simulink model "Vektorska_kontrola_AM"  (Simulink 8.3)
settings: Solver=ode3  StartTime=0  StopTime=Tfinalno  FixedStep=Tsim  RelTol=1e-3
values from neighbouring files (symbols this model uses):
  A1 = [-Rsigma/Lsigma 0 Lm/(Tr*Lr*Lsigma) 0; 0 -Rsigma/Lsigma 0 Lm/(Tr*Lr*Lsigma); Lm/Tr 0 -1/Tr 0; 0 Lm/Tr 0 -1/Tr]    [Vektorska_kontrola_AM_parametri.m]
  A2 = [0 1 0 0; -1 0 0 0; 0 0 0 1; 0 0 -1 0]    [Vektorska_kontrola_AM_parametri.m]
  A3 = [0 0 0 Lm/(Lr*Lsigma); 0 0 -Lm/(Lr*Lsigma) 0; 0 0 0 -1; 0 0 1 0]    [Vektorska_kontrola_AM_parametri.m]
  B = [1/Lsigma 0; 0 1/Lsigma; 0 0; 0 0]    [Vektorska_kontrola_AM_parametri.m]
  fdq = 50    [Vektorska_kontrola_AM_parametri.m]
  flux_bazno_dsp = Vbazno_dsp/wbazno_dsp    (= 0.0641171388295)    [Vektorska_kontrola_AM_parametri.m]
  fpwm = 20000    [Vektorska_kontrola_AM_parametri.m]
  Ibazno_dsp = Imax    (= 720)    [Vektorska_kontrola_AM_parametri.m]
  Imax = 720    [Vektorska_kontrola_AM_parametri.m]
  Isd_max = 100    [Vektorska_kontrola_AM_parametri.m]
  Isd_min = 12    [Vektorska_kontrola_AM_parametri.m]
  Isd_nom_fazno = sqrt(2)*25    [Vektorska_kontrola_AM_parametri.m]
  Isd_rel = Isd_nom_fazno/Ibazno_dsp    [Vektorska_kontrola_AM_parametri.m]
  Isq_rel = Isq_nom_fazno/Ibazno_dsp    [Vektorska_kontrola_AM_parametri.m]
  J = 0.001    [Vektorska_kontrola_AM_parametri.m]
  k_foc = 1.1    [Vektorska_kontrola_AM_parametri.m]
  k_rs = 1    [Vektorska_kontrola_AM_parametri.m]
  Ki_i = Kp_i* TkrozTsigma    [Vektorska_kontrola_AM_parametri.m]
  Ki_w = 50*0.03512/K    [Vektorska_kontrola_AM_parametri.m]
  Kp_i = (1-exp(-lambda*T))/(Kps*(exp(T/Tsigma)-1)*(1+n*(1-exp(-lambda*T))))    [Vektorska_kontrola_AM_parametri.m]
  Kp_w = 4*0.2027/K    [Vektorska_kontrola_AM_parametri.m]
  Lm = 0.00094    [Vektorska_kontrola_AM_parametri.m]
  Lm_rel = Lm/L_bazno_dsp    (= 10.55568)    [Vektorska_kontrola_AM_parametri.m]
  Lr = Lxr+Lm    (= 0.000968)    [Vektorska_kontrola_AM_parametri.m]
  Lsigma = Ls*sigm    (= 5.51900826446e-05)    [Vektorska_kontrola_AM_parametri.m]
  Lsigma_rel = Lsigma/L_bazno_dsp    (= 0.619754097415)    [Vektorska_kontrola_AM_parametri.m]
  Mopt = 2    [Vektorska_kontrola_AM_parametri.m]
  n_fw = 3500    [Vektorska_kontrola_AM_parametri.m]
  p = 2    [Vektorska_kontrola_AM_parametri.m]
  Rs_rel = Rs/R_bazno_dsp    (= 0.0284680851064)    [Vektorska_kontrola_AM_parametri.m]
  t1_step = 2    [Vektorska_kontrola_AM_parametri.m]
  t2_step = 4    [Vektorska_kontrola_AM_parametri.m]
  topt = 1    [Vektorska_kontrola_AM_parametri.m]
  Tpwm = 1/fpwm    (= 5e-05)    [Vektorska_kontrola_AM_parametri.m]
  Tpwm_SV = 1000    [Vektorska_kontrola_AM_parametri.m]
  Tr = Lr/Rr    (= 0.175680580762)    [Vektorska_kontrola_AM_parametri.m]
  TROUGAO_ZVEZDA = 0    [Vektorska_kontrola_AM_parametri.m]
  Tsim = Tpwm/16    (= 3.125e-06)    [Vektorska_kontrola_AM_parametri.m]
  Twreg1 = 320*Tsim    (= 0.001)    [Vektorska_kontrola_AM_parametri.m]
  ugao_dq = 0    [Vektorska_kontrola_AM_parametri.m]
  Vbazno_dsp = Vmax    (= 112.8)    [Vektorska_kontrola_AM_parametri.m]
  Vd = 30    [Vektorska_kontrola_AM_parametri.m]
  Vdc = 48    [Vektorska_kontrola_AM_parametri.m]
  Vq = 0    [Vektorska_kontrola_AM_parametri.m]
  wb1 = 3431    [Vektorska_kontrola_AM_parametri.m]
  wbazno_dsp = 879.64*2    (= 1759.28)    [Vektorska_kontrola_AM_parametri.m]
  wgr = 2*pi()*fgr    [Vektorska_kontrola_AM_parametri.m]
undefined symbols (not defined in the file or in its folder): DiscIntNeverNeededParam
libraries: simulink_extras x4, simulink x2

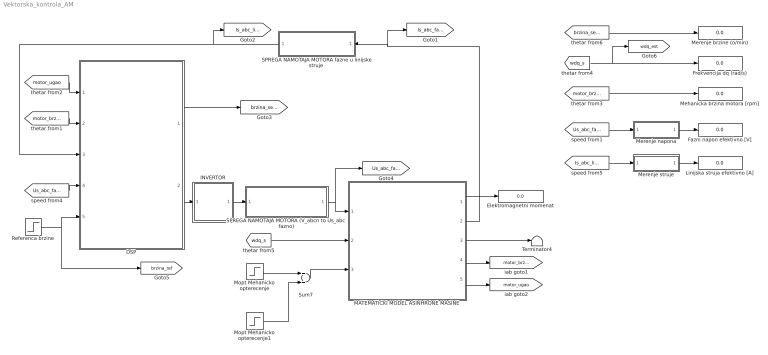
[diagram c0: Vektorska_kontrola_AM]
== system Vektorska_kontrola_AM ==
  DSP : Subsystem
  Elektromagnetni momenat : Display
  Fazni napon efektivno [V] : Display
  Frekvencija dq (rad/s) : Display
  INVERTOR : Subsystem
  Linijska struja efektivno [A] : Display
  MATEMATICKI MODEL ASINHRONE MASINE : Subsystem
  Mehanicka brzina motora [rpm] : Display
  Merenje brzine (o/min) : Display
  Merenje napona : Subsystem
  Merenje struje : Subsystem
  Mopt Mehanicko opterecenje : Step  Time=topt  After=Mopt  SampleTime=Tsim
  Mopt Mehanicko opterecenje1 : Step  Time=3*topt  After=Mopt  SampleTime=Tsim
  Referenca brzine : Step  Time=0.5  After=300  SampleTime=Tsim
  SPREGA NAMOTAJA MOTORA (V_abcn to Us_abc  fazno) : Subsystem
  "SPREGA NAMOTAJA MOTORA fazne u linijske struje " : Subsystem
  Sum7 : Sum  SampleTime=Tsim
  Terminator4 : Terminator
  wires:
  [wdq_s] -> MATEMATICKI MODEL ASINHRONE MASINE/2(W_dq)
  MATEMATICKI MODEL ASINHRONE MASINE/1(M_el) -> Elektromagnetni momenat/1
  Merenje napona/1(Us_eff) -> Fazni napon efektivno [V]/1
  Merenje struje/1(Is_eff) -> Linijska struja efektivno [A]/1
  [Is_abc_linijsko] -> Merenje struje/1(Is_abc)
  [Us_abc_fazno] -> Merenje napona/1(Us_abc)
  [motor_brzina] -> Mehanicka brzina motora [rpm]/1
  "SPREGA NAMOTAJA MOTORA fazne u linijske struje "/1("Is_abc  invertor ") -> [Is_abc_linijsko], DSP/3(Is_abc (linijsko))
  [motor_brzina] -> DSP/2(Mehanicka brzina  [o/min])
  [motor_ugao] -> DSP/1(Ugao el [rad])
  [Us_abc_fazno] -> DSP/4(Us_abc (fazno))
  INVERTOR/1(U_abcn) -> SPREGA NAMOTAJA MOTORA (V_abcn to Us_abc  fazno)/1(Uabc_prema_n)
  DSP/2(V_abc ref) -> INVERTOR/1(ABC)
  SPREGA NAMOTAJA MOTORA (V_abcn to Us_abc  fazno)/1(Us_abc_fazno) -> MATEMATICKI MODEL ASINHRONE MASINE/1(Us_abc), [Us_abc_fazno]
  [wdq_s] -> [wdq_est], Frekvencija dq (rad/s)/1
  DSP/1(Brzina (est) Senzor) -> [brzina_senzor]
  [brzina_senzor] -> Merenje brzine (o/min)/1
  MATEMATICKI MODEL ASINHRONE MASINE/2(Is_abc) -> "SPREGA NAMOTAJA MOTORA fazne u linijske struje "/1(Is_abc fazno), [Is_abc_fazno]
  Referenca brzine/1 -> DSP/5(Referenca brzine), [brzina_ref]
  MATEMATICKI MODEL ASINHRONE MASINE/5(ugao rot_el) -> [motor_ugao]
  MATEMATICKI MODEL ASINHRONE MASINE/4(Brzina meh [o/min]) -> [motor_brzina]
  Mopt Mehanicko opterecenje/1 -> Sum7/1
  Mopt Mehanicko opterecenje1/1 -> Sum7/2
  Sum7/1 -> MATEMATICKI MODEL ASINHRONE MASINE/3(Mopt)
  MATEMATICKI MODEL ASINHRONE MASINE/3(Wr_el) -> Terminator4/1

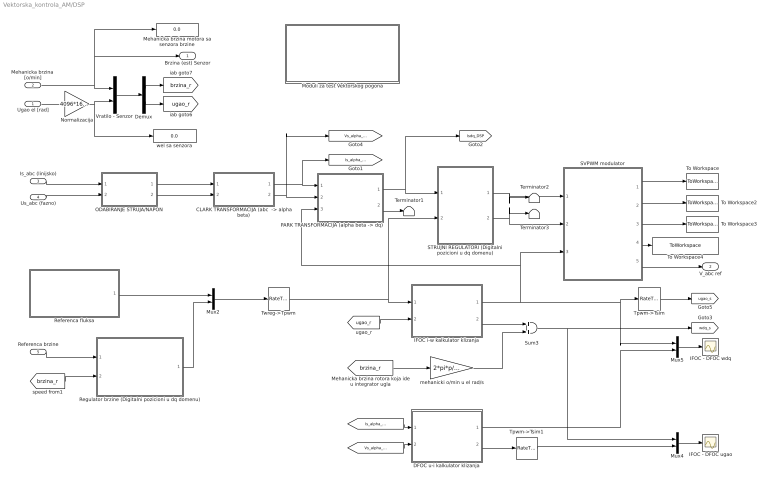
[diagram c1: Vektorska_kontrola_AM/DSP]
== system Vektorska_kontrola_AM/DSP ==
  Ugao el [rad] : Inport
  Mehanicka brzina  [o/min] : Inport  Port=2
  Is_abc (linijsko) : Inport  Port=3
  Us_abc (fazno) : Inport  Port=4
  Referenca brzine : Inport  Port=5
  "CLARK TRANSFORMACIJA (abc  -> alpha beta)" : Subsystem
  DFOC u-i kalkulator klizanja : Subsystem
  Demux : Demux  Outputs=2
  IFOC - DFOC ugao : Scope
  IFOC - DFOC wdq : Scope
  IFOC i-w kalkulator klizanja : Subsystem
  Mehanicka brzina motora sa senzora brzine : Display
  Moduli za test Vektorskog pogona : Subsystem
  Mux2 : Mux  Inputs=2
  Mux4 : Mux  Inputs=2
  Mux5 : Mux  Inputs=2
  Normalizacija : Gain  Gain=4096*16/(2*pi)  SampleTime=Tsim
  ODABIRANJE STRUJA/NAPON : Subsystem
  "PARK TRANSFORMACIJA (alpha beta -> dq)" : Subsystem
  Referenca fluksa : Subsystem
  Regulator brzine (Digitalni pozicioni u dq domenu) : Subsystem
  STRUJNI REGULATORI (Digitalni pozicioni u dq domenu) : Subsystem
  SVPWM modulator : Subsystem
  Sum3 : Sum  SampleTime=Tsim
  Terminator1 : Terminator
  Terminator2 : Terminator
  Terminator3 : Terminator
  To Workspace : ToWorkspace  VariableName=ugao  SampleTime=-1
  To Workspace2 : ToWorkspace  VariableName=BrojSektora  SampleTime=-1
  To Workspace3 : ToWorkspace  VariableName=T1T2T0  SampleTime=-1
  To Workspace4 : ToWorkspace  VariableName=LONG_MIDDLE_SHORT  SampleTime=-1
  Tpwm->Tsim : RateTransition  OutPortSampleTime=Tsim
  Tpwm->Tsim1 : RateTransition  OutPortSampleTime=Tsim
  Twreg->Tpwm : RateTransition  OutPortSampleTime=Tpwm
  Vratilo - Senzor : Mux  Inputs=2
  mehanicki o/min u el rad/s : Gain  Gain=2*pi*p/60  SampleTime=Tsim
  wel sa senzora : Display
  Brzina (est) Senzor : Outport
  V_abc ref : Outport  Port=2
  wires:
  Ugao el [rad]/1 -> Normalizacija/1
  Mehanicka brzina  [o/min]/1 -> Vratilo - Senzor/1, Mehanicka brzina motora sa senzora brzine/1, Brzina (est) Senzor/1
  Vratilo - Senzor/1 -> Demux/1
  Demux/1 -> [brzina_r]
  Normalizacija/1 -> Vratilo - Senzor/2, wel sa senzora/1
  ODABIRANJE STRUJA/NAPON/1(Is_abc DSP) -> "CLARK TRANSFORMACIJA (abc  -> alpha beta)"/1(Is_abc)
  ODABIRANJE STRUJA/NAPON/2(Us_abc DSP) -> "CLARK TRANSFORMACIJA (abc  -> alpha beta)"/2(Us_abc)
  "PARK TRANSFORMACIJA (alpha beta -> dq)"/2(Us_dq) -> Terminator1/1
  "CLARK TRANSFORMACIJA (abc  -> alpha beta)"/1(Is_alpha_beta) -> [Is_alpha_beta_DSP], "PARK TRANSFORMACIJA (alpha beta -> dq)"/1(Is_alpha_beta)
  "CLARK TRANSFORMACIJA (abc  -> alpha beta)"/2(Us_alpha_beta) -> [Vs_alpha_beta_DSP], "PARK TRANSFORMACIJA (alpha beta -> dq)"/2(Us_alpha_beta)
  Regulator brzine (Digitalni pozicioni u dq domenu)/1(Referenca momenta) -> Mux2/2
  Is_abc (linijsko)/1 -> ODABIRANJE STRUJA/NAPON/1(Is_abc)
  [brzina_r] -> mehanicki o/min u el rad/s/1
  [brzina_r] -> Regulator brzine (Digitalni pozicioni u dq domenu)/2(nr)
  Referenca brzine/1 -> Regulator brzine (Digitalni pozicioni u dq domenu)/1(nr_ref)
  SVPWM modulator/5(Tabc) -> V_abc ref/1
  "PARK TRANSFORMACIJA (alpha beta -> dq)"/1(Is_dq) -> [Isdq_DSP], STRUJNI REGULATORI (Digitalni pozicioni u dq domenu)/1(Is_dq)
  Us_abc (fazno)/1 -> ODABIRANJE STRUJA/NAPON/2(Us_abc)
  Mux2/1 -> Twreg->Tpwm/1
  SVPWM modulator/4(LONG_MIDDLE_SHORT) -> To Workspace4/1
  SVPWM modulator/3(T1T2T0) -> To Workspace3/1
  SVPWM modulator/2(BrojSektora) -> To Workspace2/1
  SVPWM modulator/1(ugao) -> To Workspace/1
  Referenca fluksa/1(Flux_referenca) -> Mux2/1
  Demux/2 -> [ugao_r]
  Tpwm->Tsim/1 -> [ugao_s]
  STRUJNI REGULATORI (Digitalni pozicioni u dq domenu)/1(Vds_ref) -> SVPWM modulator/1(Vsd_ref), Terminator2/1
  STRUJNI REGULATORI (Digitalni pozicioni u dq domenu)/2(Vqs_ref) -> SVPWM modulator/2(Vsq_ref), Terminator3/1
  IFOC i-w kalkulator klizanja/1(ugao) -> "PARK TRANSFORMACIJA (alpha beta -> dq)"/3(ugao_DSP), SVPWM modulator/3(ugao dq), Mux5/1, Tpwm->Tsim/1
  IFOC i-w kalkulator klizanja/2(w_k) -> Sum3/1
  Mux4/1 -> IFOC - DFOC ugao/1
  DFOC u-i kalkulator klizanja/2(w_dq) -> Tpwm->Tsim1/1
  Sum3/1 -> [wdq_s], Mux4/1
  Mux5/1 -> IFOC - DFOC wdq/1
  Twreg->Tpwm/1 -> STRUJNI REGULATORI (Digitalni pozicioni u dq domenu)/2(Is_dq_ref), IFOC i-w kalkulator klizanja/1(Is_dq_ref)
  [ugao_r] -> IFOC i-w kalkulator klizanja/2(ugao rotor)
  mehanicki o/min u el rad/s/1 -> Sum3/2
  [Is_alpha_beta_DSP] -> DFOC u-i kalkulator klizanja/1(Is_alpha_beta)
  [Vs_alpha_beta_DSP] -> DFOC u-i kalkulator klizanja/2(Us_alpha_beta)
  Tpwm->Tsim1/1 -> Mux4/2
  DFOC u-i kalkulator klizanja/1(ugao) -> Mux5/2

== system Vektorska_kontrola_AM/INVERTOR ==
  ABC : Inport
  Pojacanje : Gain  Gain=2/Tpwm_SV
  Proizvod : Product
  U_abcn : Outport  InitialOutput=0
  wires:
  Pojacanje/1 -> U_abcn/1
  [DC_napon] -> Proizvod/2
  ABC/1 -> Proizvod/1
  Proizvod/1 -> Pojacanje/1

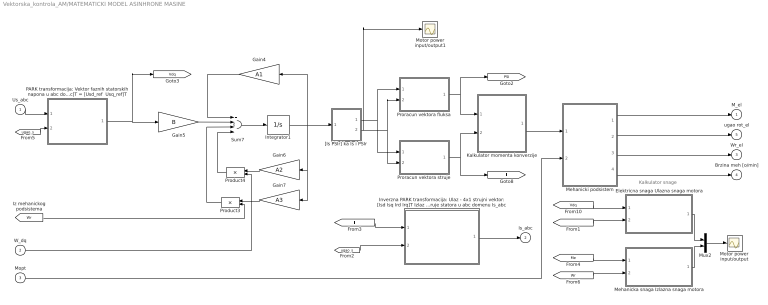
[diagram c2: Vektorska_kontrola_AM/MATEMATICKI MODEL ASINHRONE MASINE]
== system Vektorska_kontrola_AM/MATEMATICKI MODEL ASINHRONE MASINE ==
  note: Kalkulator snage
  Us_abc : Inport
  W_dq : Inport  Port=2
  Mopt : Inport  Port=3
  Elektricna snaga Ulazna snaga motora : Subsystem
  Gain4 : Gain  Gain=A1  Multiplication=Matrix(K*u) (u vector)  SampleTime=Tsim
  Gain5 : Gain  Gain=B  Multiplication=Matrix(K*u) (u vector)  SampleTime=Tsim
  Gain6 : Gain  Gain=A2  Multiplication=Matrix(K*u) (u vector)  SampleTime=Tsim
  Gain7 : Gain  Gain=A3  Multiplication=Matrix(K*u) (u vector)  SampleTime=Tsim
  Integrator1 : Integrator  InitialCondition=[0,0,0,0]
  Inverzna PARK transformacija: Ulaz - 4x1 strujni vektor: [Isd Isq Ird Irq]T Izlaz - vektor struje statora u abc domenu Is_abc : Subsystem
  Kalkulator momenta konverzije : Subsystem
  Mehanicka snaga Izlazna snaga motora : Subsystem
  Mehanicki podsistem : Subsystem
  Motor power input/output : Scope
  Motor power input/output1 : Scope
  Mux2 : Mux  Inputs=2
  PARK transformacija: Vektor faznih statorskih napona u abc domenu u vektor napona u dq referentnom sistemu - [Usa  Usb Usc]T = [Usd_ref  Usq_ref]T : Subsystem
  Product3 : Product  SampleTime=Tsim
  Product4 : Product  SampleTime=Tsim
  Proracun vektora fluksa : Subsystem
  Proracun vektora struje : Subsystem
  Sum7 : Sum  Inputs=++++  SampleTime=Tsim
  "[Is PSIr] ka Is i PSIr" : Subsystem
  M_el : Outport  InitialOutput=0
  Is_abc : Outport  Port=2  InitialOutput=0
  Wr_el : Outport  Port=3  InitialOutput=0
  Brzina meh [o/min] : Outport  Port=4  InitialOutput=0
  ugao rot_el : Outport  Port=5  InitialOutput=0
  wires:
  Us_abc/1 -> PARK transformacija: Vektor faznih statorskih napona u abc domenu u vektor napona u dq referentnom sistemu - [Usa  Usb Usc]T = [Usd_ref  Usq_ref]T/1(Us_abc)
  [ugao_s] -> PARK transformacija: Vektor faznih statorskih napona u abc domenu u vektor napona u dq referentnom sistemu - [Usa  Usb Usc]T = [Usd_ref  Usq_ref]T/2(ugao_dq)
  Integrator1/1 -> Gain4/1, Gain7/1, Gain6/1, "[Is PSIr] ka Is i PSIr"/1(X1)
  [Wr] -> Product3/2
  Product3/1 -> Sum7/3
  Gain7/1 -> Product3/1
  Gain6/1 -> Product4/1
  Sum7/1 -> Integrator1/1
  Gain4/1 -> Sum7/1
  Gain5/1 -> Sum7/2
  W_dq/1 -> Product4/2
  [ugao_s] -> Inverzna PARK transformacija: Ulaz - 4x1 strujni vektor: [Isd Isq Ird Irq]T Izlaz - vektor struje statora u abc domenu Is_abc/2(ugao_dq)
  [I] -> Inverzna PARK transformacija: Ulaz - 4x1 strujni vektor: [Isd Isq Ird Irq]T Izlaz - vektor struje statora u abc domenu Is_abc/1(I)
  PARK transformacija: Vektor faznih statorskih napona u abc domenu u vektor napona u dq referentnom sistemu - [Usa  Usb Usc]T = [Usd_ref  Usq_ref]T/1(Us_dq) -> Gain5/1, [Vdq]
  Inverzna PARK transformacija: Ulaz - 4x1 strujni vektor: [Isd Isq Ird Irq]T Izlaz - vektor struje statora u abc domenu Is_abc/1(Is_abc) -> Is_abc/1
  [I] -> Elektricna snaga Ulazna snaga motora/2(Is_dq)
  Elektricna snaga Ulazna snaga motora/1(Pel) -> Mux2/1
  [Me] -> Mehanicka snaga Izlazna snaga motora/1(Me)
  [Wr] -> Mehanicka snaga Izlazna snaga motora/2(Wr)
  Mux2/1 -> Motor power input/output/1
  Mehanicka snaga Izlazna snaga motora/1(Pmeh) -> Mux2/2
  [Vdq] -> Elektricna snaga Ulazna snaga motora/1(Vs_dq)
  Product4/1 -> Sum7/4
  "[Is PSIr] ka Is i PSIr"/1(Is) -> Proracun vektora struje/1(Is), Proracun vektora fluksa/1(Is)
  "[Is PSIr] ka Is i PSIr"/2(PSIr) -> Motor power input/output1/1, Proracun vektora struje/2(PSIr), Proracun vektora fluksa/2(PSIr)
  Proracun vektora fluksa/1(PSI) -> [PSI], Kalkulator momenta konverzije/1(PSI)
  Proracun vektora struje/1(I) -> [I], Kalkulator momenta konverzije/2(I)
  Kalkulator momenta konverzije/1(Me) -> Mehanicki podsistem/1(Mel)
  Mopt/1 -> Mehanicki podsistem/2(Mopt)
  Mehanicki podsistem/1(Me) -> M_el/1
  Mehanicki podsistem/2(ugao rot_el) -> ugao rot_el/1
  Mehanicki podsistem/3(Wr_el) -> Wr_el/1
  Mehanicki podsistem/4(Brzina meh [o/min]) -> Brzina meh [o/min]/1

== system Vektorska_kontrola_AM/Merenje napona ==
  Us_abc : Inport
  Mux : Mux  Inputs=2
  Us_alfa : Fcn  Expr=(2/3)*(u[1]-(u[2]+u[3])/2)  SampleTime=Tsim
  Us_amplituda : Fcn  Expr=sqrt(u[1]^2+u[2]^2)  SampleTime=Tsim
  Us_beta : Fcn  Expr=(u[2]-u[3])/sqrt(3)  SampleTime=Tsim
  Us_eff : Outport
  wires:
  Us_abc/1 -> Us_beta/1, Us_alfa/1
  Us_alfa/1 -> Mux/1
  Us_beta/1 -> Mux/2
  Mux/1 -> Us_amplituda/1
  Us_amplituda/1 -> Us_eff/1

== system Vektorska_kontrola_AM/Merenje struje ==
  Is_abc : Inport
  Is_alfa : Fcn  Expr=(2/3)*(u[1]-(u[2]+u[3])/2)  SampleTime=Tsim
  Is_amplituda : Fcn  Expr=sqrt(u[1]^2+u[2]^2)/sqrt(2)  SampleTime=Tsim
  Is_beta : Fcn  Expr=(u[2]-u[3])/sqrt(3)  SampleTime=Tsim
  Mux : Mux  Inputs=2
  Is_eff : Outport
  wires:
  Is_amplituda/1 -> Is_eff/1
  Mux/1 -> Is_amplituda/1
  Is_beta/1 -> Mux/2
  Is_alfa/1 -> Mux/1
  Is_abc/1 -> Is_alfa/1, Is_beta/1

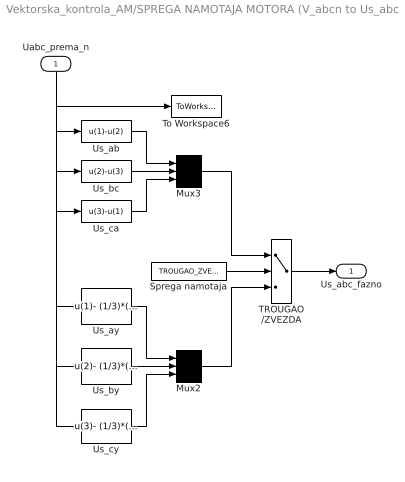
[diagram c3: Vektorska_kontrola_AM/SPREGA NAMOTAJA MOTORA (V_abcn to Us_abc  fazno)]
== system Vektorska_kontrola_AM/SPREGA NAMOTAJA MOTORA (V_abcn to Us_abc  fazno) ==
  Uabc_prema_n : Inport
  Mux2 : Mux  Inputs=3
  Mux3 : Mux  Inputs=3
  Sprega namotaja : Constant  Value=TROUGAO_ZVEZDA  SampleTime=Tsim
  TROUGAO /ZVEZDA : Switch  Threshold=0.1  SampleTime=Tsim
  To Workspace6 : ToWorkspace  VariableName=U_abc_n  SampleTime=Tsim
  Us_ab : Fcn  Expr=u(1)-u(2)  SampleTime=Tsim
  Us_ay : Fcn  Expr=u(1)- (1/3)*(u(1)+u(2)+u(3))  SampleTime=Tsim
  Us_bc : Fcn  Expr=u(2)-u(3)  SampleTime=Tsim
  Us_by : Fcn  Expr=u(2)- (1/3)*(u(1)+u(2)+u(3))  SampleTime=Tsim
  Us_ca : Fcn  Expr=u(3)-u(1)  SampleTime=Tsim
  Us_cy : Fcn  Expr=u(3)- (1/3)*(u(1)+u(2)+u(3))  SampleTime=Tsim
  Us_abc_fazno : Outport  InitialOutput=0
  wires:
  Uabc_prema_n/1 -> Us_ab/1, Us_bc/1, Us_ca/1, Us_ay/1, Us_cy/1, Us_by/1, To Workspace6/1
  Us_by/1 -> Mux2/2
  Us_cy/1 -> Mux2/3
  Us_ay/1 -> Mux2/1
  Us_ab/1 -> Mux3/1
  Us_bc/1 -> Mux3/2
  Us_ca/1 -> Mux3/3
  Mux3/1 -> TROUGAO /ZVEZDA/1
  Mux2/1 -> TROUGAO /ZVEZDA/3
  TROUGAO /ZVEZDA/1 -> Us_abc_fazno/1
  Sprega namotaja/1 -> TROUGAO /ZVEZDA/2

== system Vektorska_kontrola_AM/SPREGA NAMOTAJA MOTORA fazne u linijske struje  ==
  Is_abc fazno : Inport
  Isa_lin=Isa-Isc : Fcn  Expr=u(1)-u(3)  SampleTime=Tsim
  Isb_lin=Isb-Isa : Fcn  Expr=u(2)-u(1)  SampleTime=Tsim
  Isc_lin=Isc-Isb : Fcn  Expr=u(3)-u(2)  SampleTime=Tsim
  Mux2 : Mux  Inputs=3
  Sprega namotaja : Constant  Value=TROUGAO_ZVEZDA
  TROUGAO/ZVEZDA : Switch  Threshold=0.1  SampleTime=Tsim
  "Is_abc  invertor " : Outport  InitialOutput=0
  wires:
  Isc_lin=Isc-Isb/1 -> Mux2/3
  Isb_lin=Isb-Isa/1 -> Mux2/2
  Isa_lin=Isa-Isc/1 -> Mux2/1
  Is_abc fazno/1 -> Isc_lin=Isc-Isb/1, Isb_lin=Isb-Isa/1, Isa_lin=Isa-Isc/1, TROUGAO/ZVEZDA/3
  TROUGAO/ZVEZDA/1 -> "Is_abc  invertor "/1
  Mux2/1 -> TROUGAO/ZVEZDA/1
  Sprega namotaja/1 -> TROUGAO/ZVEZDA/2

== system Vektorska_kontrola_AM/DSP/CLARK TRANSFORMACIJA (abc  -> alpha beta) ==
  Is_abc : Inport
  Us_abc : Inport  Port=2
  Is_alfa : Fcn  Expr=2/3*(u[1]-(u[2]+u[3])/2)
  Is_beta : Fcn  Expr=(u[2]-u[3])/sqrt(3)
  Mux : Mux  Inputs=2
  Mux1 : Mux  Inputs=2
  Us_alfa : Fcn  Expr=(2/3)*(u[1]-(u[2]+u[3])/2)
  Us_beta : Fcn  Expr=(u[2]-u[3])/sqrt(3)
  Is_alpha_beta : Outport
  Us_alpha_beta : Outport  Port=2
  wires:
  Is_beta/1 -> Mux1/2
  Is_alfa/1 -> Mux1/1
  Mux1/1 -> Is_alpha_beta/1
  Mux/1 -> Us_alpha_beta/1
  Us_beta/1 -> Mux/2
  Us_alfa/1 -> Mux/1
  Us_abc/1 -> Us_beta/1, Us_alfa/1
  Is_abc/1 -> Is_beta/1, Is_alfa/1

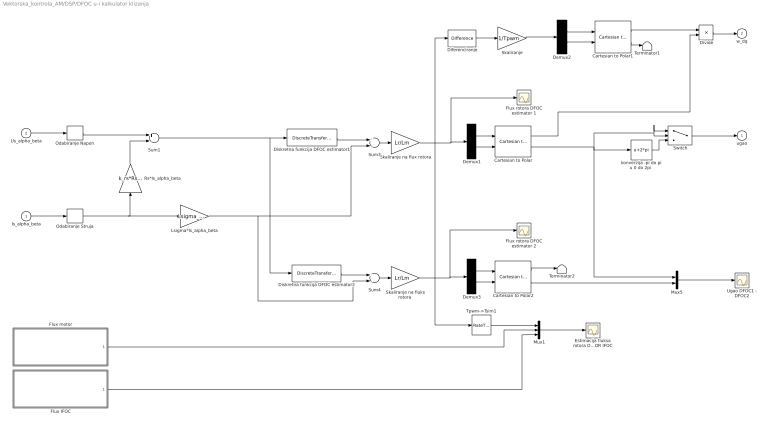
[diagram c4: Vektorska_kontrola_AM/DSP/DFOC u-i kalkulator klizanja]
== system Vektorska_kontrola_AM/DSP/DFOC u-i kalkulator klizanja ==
  Is_alpha_beta : Inport
  Us_alpha_beta : Inport  Port=2
  Cartesian to Polar : simulink_extras/Transformations/Cartesian to Polar
  Cartesian to Polar1 : simulink_extras/Transformations/Cartesian to Polar
  Cartesian to Polar2 : simulink_extras/Transformations/Cartesian to Polar
  Demux1 : Demux  Outputs=2
  Demux2 : Demux  Outputs=2
  Demux3 : Demux  Outputs=2
  Diferenciranje : simulink/Discrete/Difference  ICPrevInput=0.0  OutMin=[]  OutMax=[]  OutDataType=fixdt(1, 16)  OutScaling=2^-10  DoSatur=off
  Diskretna funkcija DFOC estimator1 : DiscreteTransferFcn  Numerator=[wbazno_dsp*Tpwm]  Denominator=[1 -(1-wgr*Tpwm)]  SampleTime=Tpwm
  Diskretna funkcija DFOC estimator2 : DiscreteTransferFcn  Numerator=[wbazno_dsp*Tpwm]  Denominator=[1 -1]  SampleTime=Tpwm
  Divide : Product  Inputs=*/  SampleTime=Tpwm
  Estimacija fluksa rotora DFOC MOTOR IFOC : Scope
  Flux IFOC : Subsystem
  Flux motor : Subsystem
  Flux rotora DFOC estimator 1 : Scope
  Flux rotora DFOC estimator 2 : Scope
  Lsigma*Is_alpha_beta : Gain  Gain=Lsigma_rel  SampleTime=Tpwm
  Mux1 : Mux  Inputs=3
  Mux5 : Mux  Inputs=2
  Odabiranje Napon : ZeroOrderHold  SampleTime=Tpwm
  Odabiranje Struja : ZeroOrderHold  SampleTime=Tpwm
  Rs*Is_alpha_beta : Gain  Gain=k_rs*Rs_rel  SampleTime=Tpwm
  Skaliranje : Gain  Gain=1/Tpwm  SampleTime=Tpwm
  "Skaliranje na fluks rotora " : Gain  Gain=Lr/Lm  SampleTime=Tpwm
  Skaliranje na flux rotora : Gain  Gain=Lr/Lm  SampleTime=Tpwm
  Sum1 : Sum  Inputs=+-  SampleTime=Tpwm
  Sum3 : Sum  Inputs=+-  SampleTime=Tpwm
  Sum4 : Sum  Inputs=+-  SampleTime=Tpwm
  Switch : Switch
  Terminator1 : Terminator
  Terminator2 : Terminator
  Tpwm->Tsim1 : RateTransition  OutPortSampleTime=Tsim
  Ugao DFOC1 - DFOC2 : Scope
  "konverzija -pi do pi u 0 do 2pi " : Fcn  Expr=u+2*pi
  ugao : Outport  InitialOutput=0
  w_dq : Outport  Port=2  InitialOutput=0
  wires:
  Switch/1 -> ugao/1
  Us_alpha_beta/1 -> Odabiranje Napon/1
  Is_alpha_beta/1 -> Odabiranje Struja/1
  Odabiranje Napon/1 -> Sum1/1
  Odabiranje Struja/1 -> Lsigma*Is_alpha_beta/1, Rs*Is_alpha_beta/1
  Rs*Is_alpha_beta/1 -> Sum1/2
  Diskretna funkcija DFOC estimator1/1 -> Sum3/1
  Lsigma*Is_alpha_beta/1 -> Sum4/2, Sum3/2
  Sum3/1 -> Skaliranje na flux rotora/1
  Demux1/1 -> Cartesian to Polar/1
  Demux1/2 -> Cartesian to Polar/2
  Skaliranje na flux rotora/1 -> Flux rotora DFOC estimator 1/1, Demux1/1, Tpwm->Tsim1/1, Diferenciranje/1
  Cartesian to Polar/2 -> "konverzija -pi do pi u 0 do 2pi "/1, Switch/2, Switch/1, Mux5/1
  "konverzija -pi do pi u 0 do 2pi "/1 -> Switch/3
  Skaliranje/1 -> Demux2/1
  Demux2/1 -> Cartesian to Polar1/1
  Demux2/2 -> Cartesian to Polar1/2
  Cartesian to Polar1/1 -> Divide/1
  Divide/1 -> w_dq/1
  Diferenciranje/1 -> Skaliranje/1
  Cartesian to Polar/1 -> Divide/2
  Sum4/1 -> "Skaliranje na fluks rotora "/1
  Diskretna funkcija DFOC estimator2/1 -> Sum4/1
  "Skaliranje na fluks rotora "/1 -> Demux3/1, Flux rotora DFOC estimator 2/1
  Demux3/1 -> Cartesian to Polar2/1
  Demux3/2 -> Cartesian to Polar2/2
  Cartesian to Polar2/2 -> Mux5/2
  Mux5/1 -> Ugao DFOC1 - DFOC2/1
  Mux1/1 -> Estimacija fluksa rotora DFOC MOTOR IFOC/1
  Tpwm->Tsim1/1 -> Mux1/1
  Cartesian to Polar1/2 -> Terminator1/1
  Cartesian to Polar2/1 -> Terminator2/1
  Sum1/1 -> Diskretna funkcija DFOC estimator2/1, Diskretna funkcija DFOC estimator1/1
  Flux motor/1(Flux motor) -> Mux1/2
  Flux IFOC/1(Flux IFOC) -> Mux1/3

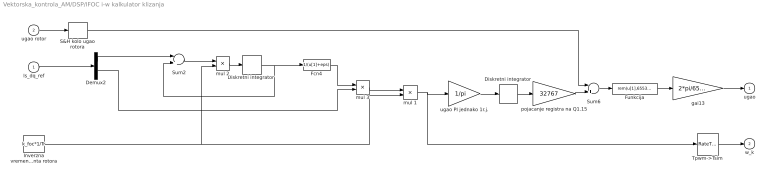
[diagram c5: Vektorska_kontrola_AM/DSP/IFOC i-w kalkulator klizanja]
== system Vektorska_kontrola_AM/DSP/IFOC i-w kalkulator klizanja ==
  Is_dq_ref : Inport
  ugao rotor : Inport  Port=2
  Demux2 : Demux  Outputs=2
  Diskretni integrator : DiscreteIntegrator  SampleTime=Tpwm  ICPrevOutput=DiscIntNeverNeededParam  ICPrevScaledInput=DiscIntNeverNeededParam
  "Diskretni integrator " : DiscreteIntegrator  SampleTime=Tpwm  ICPrevOutput=DiscIntNeverNeededParam  ICPrevScaledInput=DiscIntNeverNeededParam
  Fcn4 : Fcn  Expr=1/(u[1]+eps)  SampleTime=Tpwm
  Funkcija : Fcn  Expr=rem(u[1],65536)  SampleTime=Tpwm
  Inverzna vremenska konstanta rotora : Constant  Value=k_foc*1/Tr  SampleTime=Tpwm
  S&H kolo ugao rotora : ZeroOrderHold  SampleTime=Tpwm
  Sum2 : Sum  Inputs=|+-  SampleTime=Tpwm
  Sum6 : Sum  Inputs=|++  SampleTime=Tpwm
  Tpwm->Tsim : RateTransition  OutPortSampleTime=Tsim
  gai13 : Gain  Gain=2*pi/65535  SampleTime=Tpwm
  mul 1 : Product  SampleTime=Tpwm
  mul 2 : Product  SampleTime=Tpwm
  mul 3 : Product  SampleTime=Tpwm
  pojacanje registra na Q1.15 : Gain  Gain=32767  SampleTime=Tpwm
  ugao PI jednako 1r.j. : Gain  Gain=1/pi  SampleTime=Tpwm
  ugao : Outport  InitialOutput=0
  w_k : Outport  Port=2  InitialOutput=0
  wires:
  Fcn4/1 -> mul 3/1
  Demux2/1 -> Sum2/1
  Demux2/2 -> mul 3/2
  pojacanje registra na Q1.15/1 -> Sum6/2
  Funkcija/1 -> gai13/1
  Sum6/1 -> Funkcija/1
  mul 1/1 -> ugao PI jednako 1r.j./1, Tpwm->Tsim/1
  ugao rotor/1 -> S&H kolo ugao rotora/1
  ugao PI jednako 1r.j./1 -> Diskretni integrator/1
  Diskretni integrator/1 -> pojacanje registra na Q1.15/1
  Is_dq_ref/1 -> Demux2/1
  gai13/1 -> ugao/1
  mul 3/1 -> mul 1/1
  mul 2/1 -> "Diskretni integrator "/1
  "Diskretni integrator "/1 -> Sum2/2, Fcn4/1
  Sum2/1 -> mul 2/1
  Tpwm->Tsim/1 -> w_k/1
  S&H kolo ugao rotora/1 -> Sum6/1
  Inverzna vremenska konstanta rotora/1 -> mul 2/2, mul 1/2

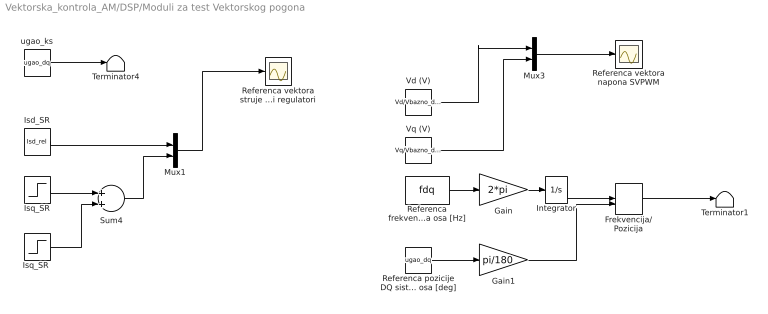
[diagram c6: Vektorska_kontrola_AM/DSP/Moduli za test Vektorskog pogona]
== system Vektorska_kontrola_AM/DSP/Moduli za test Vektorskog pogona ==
  Frekvencija/ Pozicija : ManualSwitch
  Gain : Gain  Gain=2*pi
  Gain1 : Gain  Gain=pi/180
  Integrator : Integrator
  Isd_SR : Constant  Value=Isd_rel  SampleTime=Tpwm
  Isq_SR : Step  Time=t1_step  After=Isq_rel  SampleTime=Tpwm
  "Isq_SR " : Step  Time=t2_step  After=Isq_rel  SampleTime=Tpwm
  Mux1 : Mux  Inputs=2
  Mux3 : Mux  Inputs=2
  Referenca frekvencije DQ sistema osa [Hz] : Constant  Value=fdq
  Referenca pozicije DQ sistema osa [deg] : Constant  Value=ugao_dq
  Referenca vektora napona SVPWM : Scope
  Referenca vektora struje Strujni regulatori : Scope
  Sum4 : Sum  SampleTime=Tpwm
  Terminator1 : Terminator
  Terminator4 : Terminator
  Vd (V) : Constant  Value=Vd/Vbazno_dsp
  Vq (V) : Constant  Value=Vq/Vbazno_dsp
  ugao_ks : Constant  Value=ugao_dq
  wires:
  Gain/1 -> Integrator/1
  Referenca frekvencije DQ sistema osa [Hz]/1 -> Gain/1
  Integrator/1 -> Frekvencija/ Pozicija/1
  Referenca pozicije DQ sistema osa [deg]/1 -> Gain1/1
  Gain1/1 -> Frekvencija/ Pozicija/2
  Isd_SR/1 -> Mux1/1
  Mux1/1 -> Referenca vektora struje Strujni regulatori/1
  Isq_SR/1 -> Sum4/1
  "Isq_SR "/1 -> Sum4/2
  Sum4/1 -> Mux1/2
  Vd (V)/1 -> Mux3/1
  Vq (V)/1 -> Mux3/2
  ugao_ks/1 -> Terminator4/1
  Mux3/1 -> Referenca vektora napona SVPWM/1
  Frekvencija/ Pozicija/1 -> Terminator1/1

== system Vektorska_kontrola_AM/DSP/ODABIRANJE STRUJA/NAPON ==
  Is_abc : Inport
  Us_abc : Inport  Port=2
  S&H kolo naponi : ZeroOrderHold  SampleTime=Tpwm
  S&H kolo struje : ZeroOrderHold  SampleTime=Tpwm
  Skaliranje napona DSP : Gain  Gain=1/ Vbazno_dsp  SampleTime=Tpwm
  Skaliranje struja DSP : Gain  Gain=1/Ibazno_dsp  SampleTime=Tpwm
  linijske u fazne struje - softver - : Subsystem
  Is_abc DSP : Outport  InitialOutput=0
  Us_abc DSP : Outport  Port=2  InitialOutput=0
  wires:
  linijske u fazne struje - softver -/1(Is_abc  fazno) -> Is_abc DSP/1
  Skaliranje struja DSP/1 -> linijske u fazne struje - softver -/1(Is_abc lin)
  Skaliranje napona DSP/1 -> Us_abc DSP/1
  Us_abc/1 -> S&H kolo naponi/1
  Is_abc/1 -> S&H kolo struje/1
  S&H kolo struje/1 -> Skaliranje struja DSP/1
  S&H kolo naponi/1 -> Skaliranje napona DSP/1

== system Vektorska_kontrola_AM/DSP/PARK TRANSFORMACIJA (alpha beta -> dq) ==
  Is_alpha_beta : Inport
  Us_alpha_beta : Inport  Port=2
  ugao_DSP : Inport  Port=3
  ab ->dq1 : Subsystem
  "alpha beta -> dq" : Subsystem
  Is_dq : Outport
  Us_dq : Outport  Port=2
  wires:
  "alpha beta -> dq"/1(Us_dq) -> Us_dq/1
  ab ->dq1/1(Is_dq) -> Is_dq/1
  Us_alpha_beta/1 -> "alpha beta -> dq"/1(Us_alpha_beta)
  Is_alpha_beta/1 -> ab ->dq1/1(Is_alpha_beta)
  ugao_DSP/1 -> ab ->dq1/2(ugao_DSP), "alpha beta -> dq"/2(ugao_DSP)

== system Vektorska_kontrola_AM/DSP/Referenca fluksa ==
  Deljenje : Product  Inputs=*/  SampleTime=Tsim
  Limiter reference fluksa : Subsystem
  Mload_1 : Constant  Value=Isd_nom_fazno  SampleTime=Tsim
  Mload_2 : Constant  Value=n_fw  SampleTime=Tsim
  Odabiranje Flux : ZeroOrderHold  SampleTime=Twreg1
  Referenca fluksa Isd_ref : Scope
  __1 : Gain  Gain=1/Imax  SampleTime=Tsim
  mul 3 : Product  SampleTime=Tsim
  n > n_fw Ulazak u slabljenje polja  Isd_ref = Isd_ref_nom*n/n_fw : Switch  Threshold=n_fw  SampleTime=Tsim
  Flux_referenca : Outport
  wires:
  Mload_1/1 -> __1/1
  Limiter reference fluksa/1("Isd_limit ") -> Odabiranje Flux/1
  Odabiranje Flux/1 -> Flux_referenca/1
  [brzina_r] -> Deljenje/2, n > n_fw Ulazak u slabljenje polja  Isd_ref = Isd_ref_nom*n/n_fw/2
  Mload_2/1 -> Deljenje/1
  __1/1 -> mul 3/2, n > n_fw Ulazak u slabljenje polja  Isd_ref = Isd_ref_nom*n/n_fw/3
  Deljenje/1 -> mul 3/1
  mul 3/1 -> n > n_fw Ulazak u slabljenje polja  Isd_ref = Isd_ref_nom*n/n_fw/1
  n > n_fw Ulazak u slabljenje polja  Isd_ref = Isd_ref_nom*n/n_fw/1 -> Referenca fluksa Isd_ref/1, Limiter reference fluksa/1(Isd_ref)

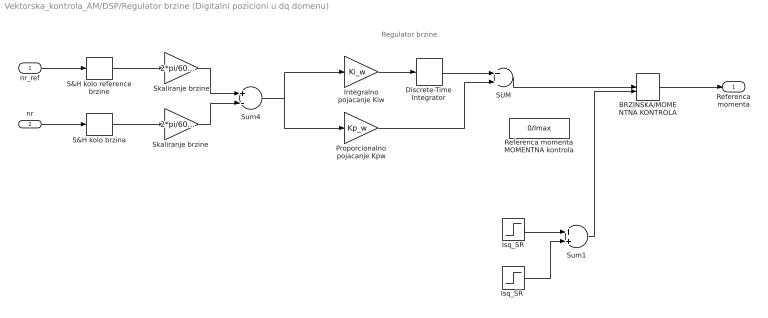
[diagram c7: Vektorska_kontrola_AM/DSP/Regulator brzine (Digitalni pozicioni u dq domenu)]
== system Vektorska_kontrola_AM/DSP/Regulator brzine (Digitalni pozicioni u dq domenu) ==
  note: Regulator brzine
  nr_ref : Inport
  nr : Inport  Port=2
  BRZINSKA/MOMENTNA KONTROLA : ManualSwitch  CurrentSetting=0
  Discrete-Time Integrator : DiscreteIntegrator  SampleTime=Twreg1  ICPrevOutput=DiscIntNeverNeededParam  ICPrevScaledInput=DiscIntNeverNeededParam
  Integralno pojacanje Kiw : Gain  Gain=Ki_w
  Isq_SR : Step  Time=t1_step  After=Isq_rel  SampleTime=Twreg1
  "Isq_SR " : Step  Time=t2_step  After=Isq_rel  SampleTime=Twreg1
  Proporcionalno pojacanje Kpw : Gain  Gain=Kp_w
  Referenca momenta MOMENTNA kontrola : Constant  Value=0/Imax  SampleTime=Twreg1
  S&H kolo brzina : ZeroOrderHold  SampleTime=Twreg1
  S&H kolo reference brzine : ZeroOrderHold  SampleTime=Twreg1
  SUM : Sum  SampleTime=Twreg1
  Skaliranje brzine : Gain  Gain=2*pi/60/wb1
  "Skaliranje brzine " : Gain  Gain=2*pi/60/wb1
  Sum1 : Sum  SampleTime=Twreg1
  Sum4 : Sum  Inputs=+-
  Referenca momenta : Outport  InitialOutput=0
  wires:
  nr/1 -> S&H kolo brzina/1
  nr_ref/1 -> S&H kolo reference brzine/1
  Skaliranje brzine/1 -> Sum4/1
  "Skaliranje brzine "/1 -> Sum4/2
  Sum4/1 -> Proporcionalno pojacanje Kpw/1, Integralno pojacanje Kiw/1
  Integralno pojacanje Kiw/1 -> Discrete-Time Integrator/1
  Discrete-Time Integrator/1 -> SUM/1
  Proporcionalno pojacanje Kpw/1 -> SUM/2
  SUM/1 -> BRZINSKA/MOMENTNA KONTROLA/1
  BRZINSKA/MOMENTNA KONTROLA/1 -> Referenca momenta/1
  S&H kolo reference brzine/1 -> Skaliranje brzine/1
  S&H kolo brzina/1 -> "Skaliranje brzine "/1
  Isq_SR/1 -> Sum1/1
  "Isq_SR "/1 -> Sum1/2
  Sum1/1 -> BRZINSKA/MOMENTNA KONTROLA/2

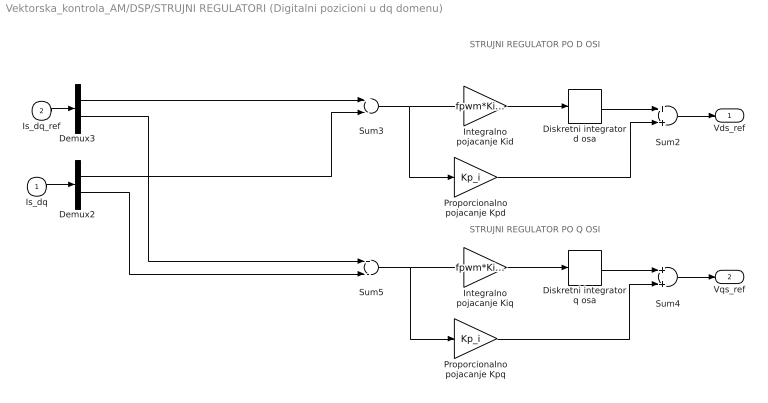
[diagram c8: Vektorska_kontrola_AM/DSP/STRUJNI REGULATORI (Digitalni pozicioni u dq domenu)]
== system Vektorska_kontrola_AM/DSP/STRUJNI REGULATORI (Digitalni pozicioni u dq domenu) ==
  note: STRUJNI REGULATOR PO D OSI
  note: STRUJNI REGULATOR PO Q OSI
  Is_dq : Inport
  Is_dq_ref : Inport  Port=2
  Demux2 : Demux  Outputs=2
  Demux3 : Demux  Outputs=2
  Diskretni integrator d osa : DiscreteIntegrator  SampleTime=Tpwm  ICPrevOutput=DiscIntNeverNeededParam  ICPrevScaledInput=DiscIntNeverNeededParam
  Diskretni integrator q osa : DiscreteIntegrator  SampleTime=Tpwm  ICPrevOutput=DiscIntNeverNeededParam  ICPrevScaledInput=DiscIntNeverNeededParam
  Integralno pojacanje Kid : Gain  Gain=fpwm*Ki_i  SampleTime=Tpwm
  Integralno pojacanje Kiq : Gain  Gain=fpwm*Ki_i  SampleTime=Tpwm
  Proporcionalno pojacanje Kpd : Gain  Gain=Kp_i  SampleTime=Tpwm
  Proporcionalno pojacanje Kpq : Gain  Gain=Kp_i  SampleTime=Tpwm
  Sum2 : Sum  SampleTime=Tpwm
  Sum3 : Sum  Inputs=+-  SampleTime=Tpwm
  Sum4 : Sum  SampleTime=Tpwm
  Sum5 : Sum  Inputs=+-  SampleTime=Tpwm
  Vds_ref : Outport  InitialOutput=0
  Vqs_ref : Outport  Port=2  InitialOutput=0
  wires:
  Is_dq/1 -> Demux2/1
  Sum3/1 -> Integralno pojacanje Kid/1, Proporcionalno pojacanje Kpd/1
  Integralno pojacanje Kid/1 -> Diskretni integrator d osa/1
  Demux2/1 -> Sum3/2
  Sum2/1 -> Vds_ref/1
  Proporcionalno pojacanje Kpd/1 -> Sum2/2
  Demux3/2 -> Sum5/1
  Demux2/2 -> Sum5/2
  Diskretni integrator d osa/1 -> Sum2/1
  Sum5/1 -> Integralno pojacanje Kiq/1, Proporcionalno pojacanje Kpq/1
  Integralno pojacanje Kiq/1 -> Diskretni integrator q osa/1
  Sum4/1 -> Vqs_ref/1
  Proporcionalno pojacanje Kpq/1 -> Sum4/2
  Diskretni integrator q osa/1 -> Sum4/1
  Is_dq_ref/1 -> Demux3/1
  Demux3/1 -> Sum3/1

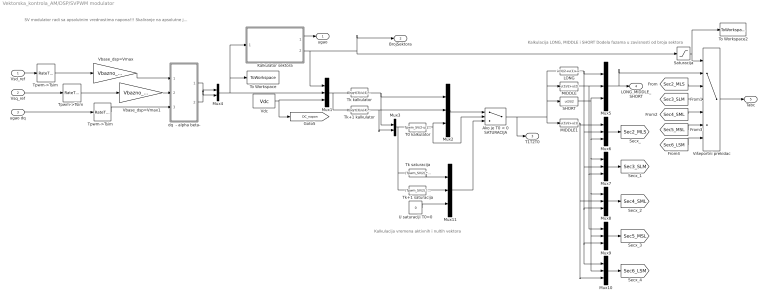
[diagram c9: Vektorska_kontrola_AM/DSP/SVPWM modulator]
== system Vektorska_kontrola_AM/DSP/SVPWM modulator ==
  note: SV modulator radi sa apsolutnim vrednostima napona!!! Skaliranje na apsolutne jedinice je neophodno
  note: Kalkulacija vremena aktivnih i nultih vektora
  note: Kalkulacija LONG, MIDDLE i SHORT Dodela fazama u zavisnosti od broja sektora
  Vsd_ref : Inport
  Vsq_ref : Inport  Port=2
  ugao dq : Inport  Port=3
  " Vbase_dsp=Vmax" : Gain  Gain=Vbazno_dsp  SampleTime=Tsim
  " Vbase_dsp=Vmax1" : Gain  Gain=Vbazno_dsp  SampleTime=Tsim
  Ako je T0 < 0 SATURACIJA : Switch
  Kalkulator sektora : Subsystem
  LONG : Fcn  Expr=u(3)/2+u(1)+u(2)
  MIDDLE : Fcn  Expr=u(3)/2+u(2)
  MIDDLE1 : Fcn  Expr=u(3)/2+u(1)
  Mux{1..2,5..11} (9 alike) : Mux  Inputs=3
  Mux3 : Mux  Inputs=2
  Mux4 : Mux  Inputs=2
  SHORT : Fcn  Expr=u(3)/2
  Saturacija : Saturate  UpperLimit=6  LowerLimit=0
  T0 kalkulator : Fcn  Expr=Tpwm_SV/2-u(1)-u(2)
  Tk kalkulator : Fcn  Expr=(sqrt(3)/u(4))*(Tpwm_SV/2)* (u(2)* sin(u(1)*pi/3)- u(3)*cos(u(1)*pi/3))
  Tk saturacija : Fcn  Expr=(Tpwm_SV/2) *u(1)/(u(1)+u(2))
  Tk+1 kalkulator : Fcn  Expr=(sqrt(3)/u(4))*(Tpwm_SV/2)* (-u(2)* sin((u(1)-1)*pi/3) + u(3)*cos((u(1)-1)*pi/3))
  Tk+1 saturacija : Fcn  Expr=(Tpwm_SV/2) *u(2)/(u(1)+u(2))
  To Workspace : ToWorkspace  VariableName=Valpha_beta  SampleTime=-1
  To Workspace2 : ToWorkspace  VariableName=BrojSektora1  SampleTime=-1
  "Tpwm->Tsim " : RateTransition  OutPortSampleTime=Tsim
  "Tpwm->Tsim  " : RateTransition  OutPortSampleTime=Tsim
  "Tpwm->Tsim   " : RateTransition  OutPortSampleTime=Tsim
  U saturaciji T0=0 : Constant  Value=0
  Vdc : Constant  Value=Vdc
  Višeportni prekidac : MultiPortSwitch  Inputs=6
  dq  - alpha beta- : Subsystem
  ugao : Outport
  BrojSektora : Outport  Port=2
  T1T2T0 : Outport  Port=3
  LONG_MIDDLE_SHORT : Outport  Port=4
  Tabc : Outport  Port=5
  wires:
  Mux4/1 -> To Workspace/1, Kalkulator sektora/1(V_alpha_beta), Mux1/2
  Kalkulator sektora/2(BrojSektora) -> BrojSektora/1, Saturacija/1, Mux1/1
  Kalkulator sektora/1(ugao) -> ugao/1
  Mux1/1 -> Tk kalkulator/1, Tk+1 kalkulator/1
  Tk kalkulator/1 -> Mux2/1, Mux3/1
  Tk+1 kalkulator/1 -> Mux2/2, Mux3/2
  Mux2/1 -> Ako je T0 < 0 SATURACIJA/1
  Mux3/1 -> T0 kalkulator/1, Tk saturacija/1, Tk+1 saturacija/1
  T0 kalkulator/1 -> Mux2/3, Ako je T0 < 0 SATURACIJA/2
  LONG/1 -> Mux5/1, Mux6/2, Mux7/2, Mux8/3, Mux9/3, Mux10/1
  MIDDLE/1 -> Mux5/2, Mux7/3, Mux9/1
  SHORT/1 -> Mux5/3, Mux6/3, Mux7/1, Mux8/1, Mux9/2, Mux10/2
  Mux5/1 -> LONG_MIDDLE_SHORT/1, Višeportni prekidac/2
  Mux6/1 -> [Sec2_MLS]
  Mux7/1 -> [Sec3_SLM]
  Mux8/1 -> [Sec4_SML]
  Mux9/1 -> [Sec5_MSL]
  Mux10/1 -> [Sec6_LSM]
  [Sec2_MLS] -> Višeportni prekidac/3
  [Sec3_SLM] -> Višeportni prekidac/4
  [Sec4_SML] -> Višeportni prekidac/5
  [Sec5_MSL] -> Višeportni prekidac/6
  [Sec6_LSM] -> Višeportni prekidac/7
  Višeportni prekidac/1 -> Tabc/1
  Saturacija/1 -> Višeportni prekidac/1, To Workspace2/1
  MIDDLE1/1 -> Mux6/1, Mux8/2, Mux10/3
  Tk+1 saturacija/1 -> Mux11/2
  Tk saturacija/1 -> Mux11/1
  Mux11/1 -> Ako je T0 < 0 SATURACIJA/3
  Ako je T0 < 0 SATURACIJA/1 -> T1T2T0/1, LONG/1, MIDDLE/1, SHORT/1, MIDDLE1/1
  U saturaciji T0=0/1 -> Mux11/3
  Vdc/1 -> [DC_napon], Mux1/3
  Vsd_ref/1 -> "Tpwm->Tsim "/1
  Vsq_ref/1 -> "Tpwm->Tsim  "/1
  ugao dq/1 -> "Tpwm->Tsim   "/1
  dq  - alpha beta-/1(Valpha_ref) -> Mux4/1
  dq  - alpha beta-/2(Vbeta_ref) -> Mux4/2
  " Vbase_dsp=Vmax"/1 -> dq  - alpha beta-/1(Vd_ref)
  " Vbase_dsp=Vmax1"/1 -> dq  - alpha beta-/2(Vq_ref)
  "Tpwm->Tsim "/1 -> " Vbase_dsp=Vmax"/1
  "Tpwm->Tsim  "/1 -> " Vbase_dsp=Vmax1"/1
  "Tpwm->Tsim   "/1 -> dq  - alpha beta-/3(ugao)

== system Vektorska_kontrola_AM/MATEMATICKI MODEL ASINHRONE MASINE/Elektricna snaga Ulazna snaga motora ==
  Vs_dq : Inport
  Is_dq : Inport  Port=2
  Demux : Demux
  Demux1 : Demux  Outputs=2
  Gain3 : Gain  Gain=3/2  SampleTime=Tsim
  Product1 : Product  SampleTime=Tsim
  Product2 : Product  SampleTime=Tsim
  Sum1 : Sum  SampleTime=Tsim
  Terminator Ird : Terminator
  Terminator Irq : Terminator
  Pel : Outport
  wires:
  Sum1/1 -> Gain3/1
  Product2/1 -> Sum1/2
  Product1/1 -> Sum1/1
  Demux/2 -> Product2/2
  Demux1/2 -> Product2/1
  Demux/1 -> Product1/2
  Demux1/1 -> Product1/1
  Demux/3 -> Terminator Ird/1
  Demux/4 -> Terminator Irq/1
  Vs_dq/1 -> Demux1/1
  Gain3/1 -> Pel/1
  Is_dq/1 -> Demux/1

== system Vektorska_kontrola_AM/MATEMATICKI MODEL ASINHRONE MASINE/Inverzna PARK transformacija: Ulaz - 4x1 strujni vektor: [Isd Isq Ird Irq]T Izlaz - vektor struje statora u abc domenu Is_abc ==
  I : Inport
  ugao_dq : Inport  Port=2
  Demux : Demux
  Is_a : Fcn  Expr=(u[1]*cos(u[3])-u[2]*sin(u[3]))  SampleTime=Tsim
  Is_b : Fcn  Expr=(u[1]*cos(u[3]-2*pi/3)-u[2]*sin(u[3]-2*pi/3))  SampleTime=Tsim
  Is_c : Fcn  Expr=(u[1]*cos(u[3]-4*pi/3)-u[2]*sin(u[3]-4*pi/3))  SampleTime=Tsim
  Mux2 : Mux  Inputs=3
  Mux3 : Mux  Inputs=3
  Terminator : Terminator
  Terminator1 : Terminator
  Is_abc : Outport
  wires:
  ugao_dq/1 -> Mux2/3
  Mux3/1 -> Is_abc/1
  I/1 -> Demux/1
  Mux2/1 -> Is_c/1, Is_a/1, Is_b/1
  Is_a/1 -> Mux3/1
  Is_b/1 -> Mux3/2
  Is_c/1 -> Mux3/3
  Demux/3 -> Terminator/1
  Demux/4 -> Terminator1/1
  Demux/1 -> Mux2/1
  Demux/2 -> Mux2/2

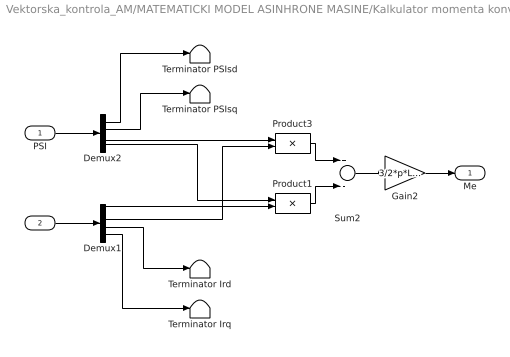
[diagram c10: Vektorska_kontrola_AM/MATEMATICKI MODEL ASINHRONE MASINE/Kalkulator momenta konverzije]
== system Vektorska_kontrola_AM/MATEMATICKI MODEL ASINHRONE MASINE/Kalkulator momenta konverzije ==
  PSI : Inport
  I : Inport  Port=2
  Demux1 : Demux
  Demux2 : Demux
  Gain2 : Gain  Gain=3/2*p*Lm/Lr  SampleTime=Tsim
  Product1 : Product  SampleTime=Tsim
  Product3 : Product  SampleTime=Tsim
  Sum2 : Sum  Inputs=+-  SampleTime=Tsim
  Terminator Ird : Terminator
  Terminator Irq : Terminator
  Terminator PSIsd : Terminator
  Terminator PSIsq : Terminator
  Me : Outport
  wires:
  PSI/1 -> Demux2/1
  Demux2/1 -> Terminator PSIsd/1
  Demux2/2 -> Terminator PSIsq/1
  Demux1/1 -> Product1/2
  Demux1/2 -> Product3/2
  I/1 -> Demux1/1
  Demux2/4 -> Product1/1
  Demux2/3 -> Product3/1
  Product3/1 -> Sum2/1
  Product1/1 -> Sum2/2
  Gain2/1 -> Me/1
  Sum2/1 -> Gain2/1
  Demux1/3 -> Terminator Ird/1
  Demux1/4 -> Terminator Irq/1

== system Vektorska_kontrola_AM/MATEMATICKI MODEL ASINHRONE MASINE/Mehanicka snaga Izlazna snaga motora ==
  note: Pmeh=Mel*Wr_el/P
  Me : Inport
  Wr : Inport  Port=2
  Gain11 : Gain  Gain=1/p  SampleTime=Tsim
  Product6 : Product  SampleTime=Tsim
  Pmeh : Outport
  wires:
  Product6/1 -> Gain11/1
  Me/1 -> Product6/1
  Gain11/1 -> Pmeh/1
  Wr/1 -> Product6/2

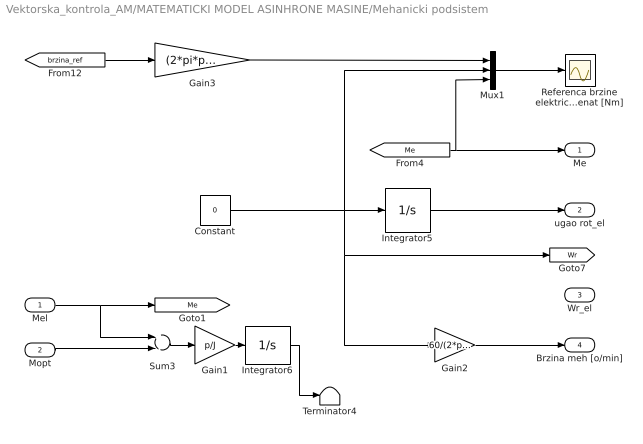
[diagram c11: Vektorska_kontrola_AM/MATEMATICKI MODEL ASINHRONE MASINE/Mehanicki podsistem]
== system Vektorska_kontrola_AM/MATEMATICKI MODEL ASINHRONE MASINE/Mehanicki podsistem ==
  Mel : Inport
  Mopt : Inport  Port=2
  Constant : Constant  Value=0  SampleTime=Tsim
  Gain1 : Gain  Gain=p/J  SampleTime=Tsim
  Gain2 : Gain  Gain=60/(2*pi*p)  SampleTime=Tsim
  Gain3 : Gain  Gain=(2*pi*p)/60  SampleTime=Tsim
  Integrator5 : Integrator
  Integrator6 : Integrator
  Mux1 : Mux  Inputs=3
  Referenca brzine elektricno [rad/s] Elektricna brzina [rad/s] Elektromagnetni momenat [Nm] : Scope
  Sum3 : Sum  Inputs=+-
  Terminator4 : Terminator
  Me : Outport
  ugao rot_el : Outport  Port=2
  Wr_el : Outport  Port=3
  Brzina meh [o/min] : Outport  Port=4
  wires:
  Mel/1 -> [Me], Sum3/1
  Integrator5/1 -> ugao rot_el/1
  Gain2/1 -> Brzina meh [o/min]/1
  Gain1/1 -> Integrator6/1
  Sum3/1 -> Gain1/1
  Mux1/1 -> Referenca brzine elektricno [rad/s] Elektricna brzina [rad/s] Elektromagnetni momenat [Nm]/1
  [brzina_ref] -> Gain3/1
  Gain3/1 -> Mux1/1
  Mopt/1 -> Sum3/2
  [Me] -> Me/1, Mux1/3
  Integrator6/1 -> Terminator4/1
  Constant/1 -> Gain2/1, [Wr], Integrator5/1, Mux1/2

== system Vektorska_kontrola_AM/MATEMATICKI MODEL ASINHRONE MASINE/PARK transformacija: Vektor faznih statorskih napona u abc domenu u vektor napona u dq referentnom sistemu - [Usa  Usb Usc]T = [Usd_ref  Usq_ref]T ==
  Us_abc : Inport
  ugao_dq : Inport  Port=2
  Demux2 : Demux  Outputs=3
  Mux : Mux
  Mux1 : Mux  Inputs=2
  Usd : Fcn  Expr=(2/3)*(u[1]*cos(u[4])+u[2]*cos(u[4]-2*pi/3)+u[3]*cos(u[4]-4*pi/3))  SampleTime=Tsim
  Usq : Fcn  Expr=-(2/3)*(u[1]*sin(u[4])+u[2]*sin(u[4]-2*pi/3)+u[3]*sin(u[4]-4*pi/3))  SampleTime=Tsim
  Us_dq : Outport
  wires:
  Usd/1 -> Mux1/1
  Usq/1 -> Mux1/2
  Mux/1 -> Usq/1, Usd/1
  Demux2/2 -> Mux/2
  Demux2/3 -> Mux/3
  Demux2/1 -> Mux/1
  ugao_dq/1 -> Mux/4
  Us_abc/1 -> Demux2/1
  Mux1/1 -> Us_dq/1

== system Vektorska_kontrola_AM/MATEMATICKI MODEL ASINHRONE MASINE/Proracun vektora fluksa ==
  Is : Inport
  PSIr : Inport  Port=2
  Gain1 : Gain  Gain=Lm/Lr  SampleTime=Tsim
  Gain4 : Gain  Gain=Lsigma  SampleTime=Tsim
  Mux1 : Mux  Inputs=2
  Sum1 : Sum  SampleTime=Tsim
  PSI : Outport
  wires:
  Is/1 -> Gain4/1
  Mux1/1 -> PSI/1
  PSIr/1 -> Gain1/1, Mux1/2
  Gain1/1 -> Sum1/2
  Gain4/1 -> Sum1/1
  Sum1/1 -> Mux1/1

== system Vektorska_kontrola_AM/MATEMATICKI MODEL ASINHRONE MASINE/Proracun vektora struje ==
  Is : Inport
  PSIr : Inport  Port=2
  Gain1 : Gain  Gain=Lm/Lr  SampleTime=Tsim
  Gain4 : Gain  Gain=1/Lr  SampleTime=Tsim
  Mux1 : Mux  Inputs=2
  Sum1 : Sum  Inputs=-+  SampleTime=Tsim
  I : Outport
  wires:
  Is/1 -> Gain1/1, Mux1/1
  Mux1/1 -> I/1
  PSIr/1 -> Gain4/1
  Gain1/1 -> Sum1/1
  Gain4/1 -> Sum1/2
  Sum1/1 -> Mux1/2

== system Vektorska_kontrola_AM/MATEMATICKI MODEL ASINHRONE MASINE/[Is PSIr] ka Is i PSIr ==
  X1 : Inport
  Demux2 : Demux
  Mux1 : Mux  Inputs=2
  Mux2 : Mux  Inputs=2
  Is : Outport
  PSIr : Outport  Port=2
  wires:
  Demux2/1 -> Mux1/1
  Demux2/4 -> Mux2/2
  X1/1 -> Demux2/1
  Mux1/1 -> Is/1
  Mux2/1 -> PSIr/1
  Demux2/3 -> Mux2/1
  Demux2/2 -> Mux1/2

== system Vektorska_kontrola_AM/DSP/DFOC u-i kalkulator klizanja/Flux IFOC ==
  Demux5 : Demux  Outputs=2
  Lm : Gain  Gain=Lm_rel  SampleTime=Tsim
  Mux2 : Mux  Inputs=2
  PSIr_q : Constant  Value=0  SampleTime=Tsim
  Terminator5 : Terminator
  Tpwm->Tsim : RateTransition  OutPortSampleTime=Tsim
  ab ->dq2 : Subsystem
  Flux IFOC : Outport
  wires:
  Mux2/1 -> ab ->dq2/1(PSIr_dq)
  PSIr_q/1 -> Mux2/2
  [ugao_s] -> ab ->dq2/2(ugao_DSP)
  Tpwm->Tsim/1 -> Lm/1
  Demux5/1 -> Tpwm->Tsim/1
  [Isdq_DSP] -> Demux5/1
  ab ->dq2/1(PSIr_alpha_beta) -> Flux IFOC/1
  Lm/1 -> Mux2/1
  Demux5/2 -> Terminator5/1

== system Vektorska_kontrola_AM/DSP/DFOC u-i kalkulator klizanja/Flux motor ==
  Demux4 : Demux
  Mux4 : Mux  Inputs=2
  Skaliranje Flux motora : Gain  Gain=1/flux_bazno_dsp  SampleTime=Tsim
  Terminator3 : Terminator
  Terminator4 : Terminator
  ab ->dq1 : Subsystem
  Flux motor : Outport
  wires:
  Demux4/4 -> Mux4/2
  Demux4/3 -> Mux4/1
  Mux4/1 -> ab ->dq1/1(PSIr_dq)
  [PSI] -> Skaliranje Flux motora/1
  Skaliranje Flux motora/1 -> Demux4/1
  [ugao_s] -> ab ->dq1/2(ugao_DSP)
  ab ->dq1/1(PSIr_alpha_beta) -> Flux motor/1
  Demux4/1 -> Terminator3/1
  Demux4/2 -> Terminator4/1

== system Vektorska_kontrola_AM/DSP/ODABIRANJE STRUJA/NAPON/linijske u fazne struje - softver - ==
  Is_abc lin : Inport
  Isa=1/3*(Isa_lin-Isb_lin) : Fcn  Expr=(1/3)* (u(1)-u(2))  SampleTime=Tpwm
  Isb=1/3*(Isb_lin-Isc_lin) : Fcn  Expr=(1/3)* (u(2)-u(3))  SampleTime=Tpwm
  Isc=1/3*(Isc_lin-Isa_lin) : Fcn  Expr=(1/3)* (u(3)-u(1))  SampleTime=Tpwm
  Mux : Mux  Inputs=3
  Sprega namotaja : Constant  Value=TROUGAO_ZVEZDA  SampleTime=Tpwm
  TROUGAO/ZVEZDA : Switch  Threshold=0.1  SampleTime=Tpwm
  Is_abc  fazno : Outport  InitialOutput=0
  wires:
  TROUGAO/ZVEZDA/1 -> Is_abc  fazno/1
  Mux/1 -> TROUGAO/ZVEZDA/1
  Isc=1/3*(Isc_lin-Isa_lin)/1 -> Mux/3
  Sprega namotaja/1 -> TROUGAO/ZVEZDA/2
  Isb=1/3*(Isb_lin-Isc_lin)/1 -> Mux/2
  Isa=1/3*(Isa_lin-Isb_lin)/1 -> Mux/1
  Is_abc lin/1 -> TROUGAO/ZVEZDA/3, Isc=1/3*(Isc_lin-Isa_lin)/1, Isb=1/3*(Isb_lin-Isc_lin)/1, Isa=1/3*(Isa_lin-Isb_lin)/1

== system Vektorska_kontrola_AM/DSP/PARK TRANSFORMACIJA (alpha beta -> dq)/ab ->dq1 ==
  Is_alpha_beta : Inport
  ugao_DSP : Inport  Port=2
  Mux12 : Mux  Inputs=2
  Mux2 : Mux  Inputs=2
  psird2 : Fcn  Expr=u(1)*cos(u(3))+u(2)*sin(u(3))
  psirq2 : Fcn  Expr=-u(1)*sin(u(3))+u(2)*cos(u(3))
  Is_dq : Outport
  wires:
  ugao_DSP/1 -> Mux12/2
  Mux2/1 -> Is_dq/1
  psird2/1 -> Mux2/1
  Mux12/1 -> psirq2/1, psird2/1
  Is_alpha_beta/1 -> Mux12/1
  psirq2/1 -> Mux2/2

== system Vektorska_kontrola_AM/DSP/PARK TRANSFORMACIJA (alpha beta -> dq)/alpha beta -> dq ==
  Us_alpha_beta : Inport
  ugao_DSP : Inport  Port=2
  Mux12 : Mux  Inputs=2
  Mux2 : Mux  Inputs=2
  psird2 : Fcn  Expr=u(1)*cos(u(3))+u(2)*sin(u(3))
  psirq2 : Fcn  Expr=-u(1)*sin(u(3))+u(2)*cos(u(3))
  Us_dq : Outport
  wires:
  psirq2/1 -> Mux2/2
  Us_alpha_beta/1 -> Mux12/1
  Mux12/1 -> psird2/1, psirq2/1
  psird2/1 -> Mux2/1
  Mux2/1 -> Us_dq/1
  ugao_DSP/1 -> Mux12/2

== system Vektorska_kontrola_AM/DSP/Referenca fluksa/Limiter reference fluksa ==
  Isd_ref : Inport
  Donji limit : Constant  Value=Isd_min/Imax  SampleTime=Tsim
  Gornji limit : Constant  Value=Isd_max/Imax  SampleTime=Tsim
  Saturacija  Fluks : simulink/Discontinuities/Saturation Dynamic  OutMin=[]  OutMax=[]  OutDataTypeStr=Inherit: Same as second input  OutDataType=fixdt(1, 16)  OutScaling=2^-10  DoSatur=off
  "Isd_limit " : Outport
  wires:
  Gornji limit/1 -> Saturacija  Fluks/1
  Isd_ref/1 -> Saturacija  Fluks/2
  Saturacija  Fluks/1 -> "Isd_limit "/1
  Donji limit/1 -> Saturacija  Fluks/3

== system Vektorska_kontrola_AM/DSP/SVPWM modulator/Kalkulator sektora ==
  V_alpha_beta : Inport
  Cartesian to Polar : simulink_extras/Transformations/Cartesian to Polar
  Demux2 : Demux  Outputs=2
  Racunanje broja sektora : Fcn  Expr=(floor(((u(1))/(2*pi))*6))+1
  Switch : Switch
  Terminator4 : Terminator
  konverzija -pi to pi : Fcn  Expr=u+2*pi
  ugao : Outport
  BrojSektora : Outport  Port=2
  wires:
  Cartesian to Polar/2 -> konverzija -pi to pi/1, Switch/2, Switch/1
  konverzija -pi to pi/1 -> Switch/3
  Switch/1 -> Racunanje broja sektora/1, ugao/1
  Racunanje broja sektora/1 -> BrojSektora/1
  V_alpha_beta/1 -> Demux2/1
  Demux2/1 -> Cartesian to Polar/1
  Demux2/2 -> Cartesian to Polar/2
  Cartesian to Polar/1 -> Terminator4/1

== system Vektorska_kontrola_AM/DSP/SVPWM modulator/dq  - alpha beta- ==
  Vd_ref : Inport
  Vq_ref : Inport  Port=2
  ugao : Inport  Port=3
  Mux12 : Mux  Inputs=2
  Mux4 : Mux  Inputs=2
  To Workspace12 : ToWorkspace  VariableName=Vdq  SampleTime=-1
  psird2 : Fcn  Expr=u(1)*cos(u(3))-u(2)*sin(u(3))
  psirq2 : Fcn  Expr=u(1)*sin(u(3))+u(2)*cos(u(3))
  Valpha_ref : Outport
  Vbeta_ref : Outport  Port=2
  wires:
  psirq2/1 -> Vbeta_ref/1
  Mux12/1 -> psird2/1, psirq2/1
  psird2/1 -> Valpha_ref/1
  ugao/1 -> Mux12/2
  Vd_ref/1 -> Mux4/1
  Mux4/1 -> Mux12/1, To Workspace12/1
  Vq_ref/1 -> Mux4/2

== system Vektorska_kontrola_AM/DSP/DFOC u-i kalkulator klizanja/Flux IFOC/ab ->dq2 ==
  PSIr_dq : Inport
  ugao_DSP : Inport  Port=2
  Mux12 : Mux  Inputs=2
  Mux2 : Mux  Inputs=2
  psird2 : Fcn  Expr=u(1)*cos(u(3))-u(2)*sin(u(3))  SampleTime=Tsim
  psirq2 : Fcn  Expr=u(1)*sin(u(3))+u(2)*cos(u(3))  SampleTime=Tsim
  PSIr_alpha_beta : Outport
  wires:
  psirq2/1 -> Mux2/2
  PSIr_dq/1 -> Mux12/1
  Mux12/1 -> psird2/1, psirq2/1
  psird2/1 -> Mux2/1
  Mux2/1 -> PSIr_alpha_beta/1
  ugao_DSP/1 -> Mux12/2

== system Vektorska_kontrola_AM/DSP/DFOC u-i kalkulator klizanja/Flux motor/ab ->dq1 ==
  PSIr_dq : Inport
  ugao_DSP : Inport  Port=2
  Mux12 : Mux  Inputs=2
  Mux2 : Mux  Inputs=2
  psird2 : Fcn  Expr=u(1)*cos(u(3))-u(2)*sin(u(3))  SampleTime=Tsim
  psirq2 : Fcn  Expr=u(1)*sin(u(3))+u(2)*cos(u(3))  SampleTime=Tsim
  PSIr_alpha_beta : Outport
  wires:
  ugao_DSP/1 -> Mux12/2
  Mux2/1 -> PSIr_alpha_beta/1
  psird2/1 -> Mux2/1
  Mux12/1 -> psirq2/1, psird2/1
  PSIr_dq/1 -> Mux12/1
  psirq2/1 -> Mux2/2
